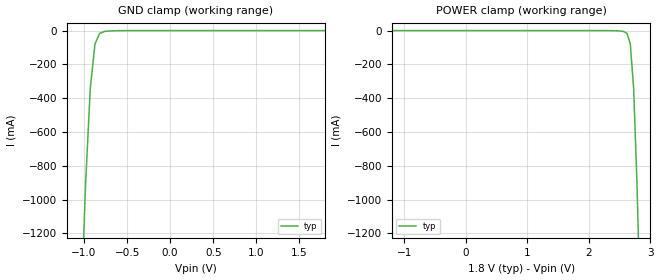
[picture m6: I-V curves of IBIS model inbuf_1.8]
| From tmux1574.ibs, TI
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| inbuf_1.8
[Model]   inbuf_1.8
Model_type   Input
Vinl = 0.45
Vinh = 1.2
|   typ   min   max
C_comp   2.533030e-12   NA   NA
[Voltage Range]   1.8   NA   NA
[Temperature Range]   27   NA   NA
[Power Clamp Reference]   1.8   NA   NA
[GND Clamp Reference]   0   NA   NA
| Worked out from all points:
|   GND clamp passes 1 mA (typ) near -0.63 V on its own axis
[GND Clamp]
|   Voltage   I(typ)   I(min)   I(max)
-3.6V     -51.95A    NA         NA
-1.036V   -1.681A    NA         NA
-981.8mV  -910.3mA   NA         NA
-927.3mV  -343.6mA   NA         NA
-872.7mV  -79.21mA   NA         NA
-818.2mV  -16.29mA   NA         NA
-763.6mV  -5.281mA   NA         NA
-545.5mV  -233.4uA   NA         NA
1.8V      300.1nA    NA         NA
[POWER Clamp]
|   Voltage   I(typ)   I(min)   I(max)
-1.8V     600.1nA    NA         NA
2.345V    -233.4uA   NA         NA
2.564V    -5.281mA   NA         NA
2.618V    -16.29mA   NA         NA
2.673V    -79.21mA   NA         NA
2.727V    -343.6mA   NA         NA
2.782V    -910.3mA   NA         NA
2.836V    -1.681A    NA         NA
3.6V      -15.98A    NA         NA
